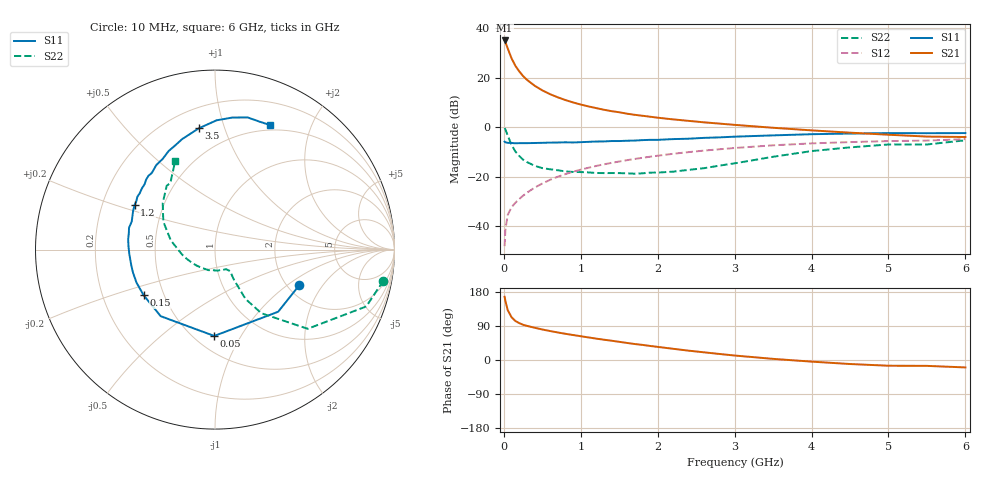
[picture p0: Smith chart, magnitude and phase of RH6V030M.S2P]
! SIEMENS Small Signal Semiconductors
! BFR106
! Si NPN RF Bipolar Junction Transistor in SOT23
! VCE = 6 V  IC = 30 mA
! Common Emitter S-Parameters:  August  1996
# GHz  S  MA  R  50
!  f  S11  S21  S12  S22
! GHz  MAG  ANG  MAG  ANG  MAG  ANG  MAG  ANG
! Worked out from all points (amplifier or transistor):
!   36 points, 10 MHz to 6 GHz, reference 50 ohm
!   highest |S21| = 35.1 dB at 10 MHz (marker M1)
!   |S21| within 3 dB of that: start of sweep to 47.73 MHz
!   unconditionally stable (mu >= 1): 303.5 MHz to 2.145 GHz
!   at 250 MHz: K = 0.95, MSG = 24.2 dB, |S12| = -27.7 dB
!   at 1.4 GHz: K = 1.06, MAG = 9.0 dB, |S12| = -14.5 dB
!   at 6 GHz: K = 0.98, MSG = 0.4 dB, |S12| = -4.8 dB
!   S11 on the Smith chart (normalised r, x): 10 MHz: 2.31, -1.24; 50 MHz: 0.62, -0.78; 150 MHz: 0.39, -0.25; 1.2 GHz: 0.34, +0.23; 3.5 GHz: 0.33, +0.82; 6 GHz: 0.44, +1.45
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0.01  0.5098 -22.9  56.91 166.8  0.0039 83.9  0.954 -10.5
0.02  0.4938 -44.5  53.11 156.0  0.0084 74.7  0.9003 -20.6
0.05  0.4811 -90.5  39.39 131.9  0.0166 62.8  0.6793 -40.5
0.1  0.4787 -129.2  24.78 112.9  0.024 56.9  0.439 -53.9
0.15  0.472 -147.3  17.45 102.9  0.0295 58.7  0.3226 -58.3
0.2  0.4744 -157.2  13.48 97.4  0.0351 62.0  0.2615 -58.1
0.25  0.4746 -164.3  10.85 93.0  0.041 63.6  0.2194 -58.0
0.3  0.4746 -169.1  9.1 90.1  0.047 65.9  0.197 -57.8
0.4  0.4781 -177.1  6.915 85.1  0.0597 67.7  0.1654 -56.3
0.5  0.4822 178.0  5.555 80.5  0.0723 69.1  0.1483 -55.3
0.6  0.4871 173.3  4.662 76.5  0.0858 69.1  0.1406 -56.2
0.7  0.489 168.9  4.027 72.7  0.0991 69.1  0.1341 -58.1
0.9  0.4896 161.4  3.164 65.9  0.1253 67.8  0.124 -60.9
1.1  0.5046 154.7  2.63 59.6  0.1509 66.0  0.1214 -69.0
1.2  0.512 151.1  2.433 56.4  0.1639 65.1  0.1183 -72.4
1.6  0.5311 140.1  1.875 45.0  0.2147 60.2  0.1162 -90.9
2.2  0.5734 124.8  1.437 29.6  0.2892 52.3  0.1257 -125.4
2.8  0.621 111.0  1.182 16.0  0.3568 43.5  0.1663 -162.3
3.5  0.6818 97.6  0.972 3.0  0.4291 33.2  0.2517 168.2
4.5  0.7421 82.5  0.774 -10.6  0.4984 18.0  0.39 138.3
5.5  0.7548 70.4  0.645 -15.5  0.535 7.8  0.4463 123.9
6  0.7593 66.0  0.632 -19.6  0.5722 0.4  0.5422 114.1
